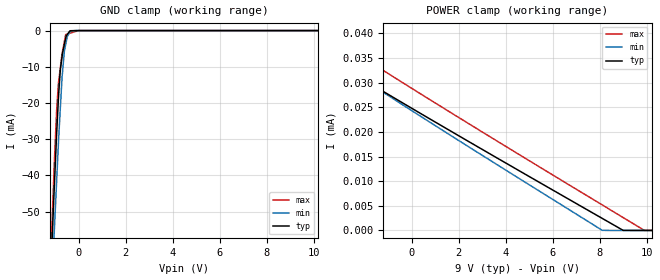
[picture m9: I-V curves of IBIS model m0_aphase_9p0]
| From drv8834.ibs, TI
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|   m0_aphase_9p0 Model
[Model]   m0_aphase_9p0
Model_type   Input
Vinl = 0.7
Vinh = 2
|   typ   min   max
|   (nom PVT)   (fast PVT)   (slow PVT)
|C_comp from frequency sweep method (F=250KHz)
|Average
|C_comp   2.754e-12   2.547e-12   2.970e-12
|C_comp from LC tank measurement(L=1nH)
|Average
|Resonant Frequency(Hz)   4.480e+09   4.560e+09   4.400e+09
 C_comp   1.263e-12   1.219e-12   1.310e-12
| Where nom  PVT is Nominal Process, 9V, 27C
|   Fast PVT is Strong Process,  9.9V, -40C
|   Slow PVT is Weak Process,   8.1V, 125C
[Voltage Range]   9   8.1   9.9
|Ambient Temperature   25   150   -40
|Junction Temperature
[Temperature Range]   27   125   -40
[Power Clamp Reference]   9   8.1   9.9
[GND Clamp Reference]   0   0   0
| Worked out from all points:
|   GND clamp passes 1 mA (typ) near -0.47 V on its own axis
[GND Clamp]
|   Voltage   I(typ)   I(min)   I(max)
-9V       -1.598A    -1.486A    -1.684A
-1.197V   -69.78mA   -80.18mA   -65.58mA
-1.053V   -46.77mA   -58.72mA   -40.68mA
-1.03V    -43.3mA    -55.38mA   -36.76mA
-930.6mV  -28.66mA   -41.72mA   -22.23mA
-861.3mV  -19.75mA   -32.17mA   -15.18mA
-765mV    -10.45mA   -20.54mA   -9.84mA
-696.6mV  -7.114mA   -12.72mA   -6.303mA
-599.4mV  -3.789mA   -5.581mA   -2.969mA
-544.5mV  -2.139mA   -3.838mA   -1.085mA
-360mV    -46.1uA    -328.8uA   -717.6uA
18V       0A         0A         0A
[POWER Clamp]
|   Voltage   I(typ)   I(min)   I(max)
-9V       4.199mA    4.225mA    5.783mA
-2.831V   219.2uA    377.2uA    44.91uA
-2.772V   182.2uA    341.8uA    37.79uA
-2.583V   78.38uA    233uA      36.86uA
-2.475V   39.05uA    171.1uA    36.33uA
-2.394V   32.08uA    127.8uA    36.08uA
-2.187V   31.02uA    42.58uA    35.45uA
-2.106V   30.79uA    32.56uA    35.21uA
-2.033V   30.58uA    30.85uA    34.99uA
8.092V    2.483uA    31.12nA    5.219uA
9.89V     0A         0A         28.54nA
18V       0A         0A         0A
